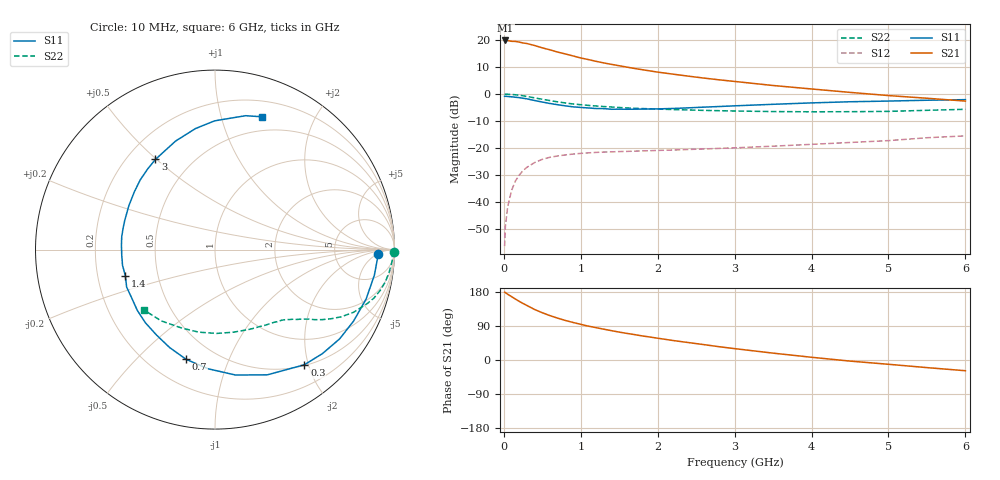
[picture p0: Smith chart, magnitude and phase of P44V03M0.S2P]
! SIEMENS Small Signal Semiconductors
! BFP182
! Si NPN RF Bipolar Junction Transistor in SOT143
! VCE = 4 V  IC = 3 mA
! Common Emitter S-Parameters:  March  1996
# GHz  S  MA  R  50
!  f  S11  S21  S12  S22
! GHz  MAG  ANG  MAG  ANG  MAG  ANG  MAG  ANG
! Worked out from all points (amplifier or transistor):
!   36 points, 10 MHz to 6 GHz, reference 50 ohm
!   highest |S21| = 19.9 dB at 20 MHz (marker M1)
!   |S21| within 3 dB of that: start of sweep to 534.5 MHz
!   unconditionally stable (mu >= 1): 1.938 GHz to 5.739 GHz
!   at 250 MHz: K = 0.15, MSG = 23.7 dB, |S12| = -28.4 dB
!   at 1.4 GHz: K = 0.78, MSG = 16.2 dB, |S12| = -21.5 dB
!   at 6 GHz: K = 0.97, MSG = 6.5 dB, |S12| = -15.6 dB
!   S11 on the Smith chart (normalised r, x): 10 MHz: 19, -6; 300 MHz: 0.51, -1.93; 700 MHz: 0.35, -0.71; 1.4 GHz: 0.32, -0.13; 3 GHz: 0.31, +0.50; 6 GHz: 0.35, +1.35
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0.01  0.9058 -1.7  9.648 178.9  0.0015 90.6  0.9946 -0.7
0.02  0.9057 -3.6  9.837 177.9  0.0035 87.0  0.989 -1.4
0.05  0.8993 -9.1  9.759 173.5  0.0081 85.9  0.9896 -3.6
0.1  0.886 -18.0  9.488 167.3  0.0162 79.6  0.9787 -7.2
0.15  0.8689 -27.2  9.442 160.8  0.0242 74.2  0.9664 -10.7
0.2  0.8542 -35.6  9.175 154.8  0.0312 70.6  0.948 -13.9
0.3  0.8121 -52.2  8.632 143.9  0.0436 61.4  0.8993 -19.6
0.4  0.7563 -67.3  7.928 133.3  0.0534 54.7  0.8466 -24.4
0.5  0.7081 -80.7  7.168 124.7  0.0613 48.1  0.7973 -28.0
0.6  0.6652 -93.3  6.592 117.1  0.067 43.4  0.7541 -30.7
0.7  0.6319 -104.8  5.984 110.4  0.0708 39.8  0.7143 -33.1
0.8  0.6013 -114.9  5.527 104.3  0.074 36.2  0.6808 -35.0
0.9  0.577 -124.3  5.074 99.0  0.0768 33.5  0.6528 -36.4
1.1  0.5497 -141.9  4.344 89.3  0.0808 29.7  0.6134 -39.2
1.4  0.5204 -163.7  3.54 77.4  0.0843 25.6  0.5731 -42.8
1.8  0.5245 172.2  2.82 63.5  0.0879 23.5  0.5362 -47.7
2.2  0.5385 153.1  2.331 51.4  0.0911 22.8  0.5139 -53.4
3  0.6023 123.4  1.708 30.0  0.1001 22.5  0.4828 -67.3
3.5  0.6432 110.0  1.436 18.1  0.1075 22.4  0.4714 -77.5
4.5  0.7172 90.2  1.07 -2.9  0.1259 21.1  0.4689 -101.3
5.5  0.7653 77.1  0.833 -20.1  0.1541 18.6  0.4974 -127.0
6  0.7843 70.7  0.738 -28.3  0.1669 15.0  0.5194 -139.5
